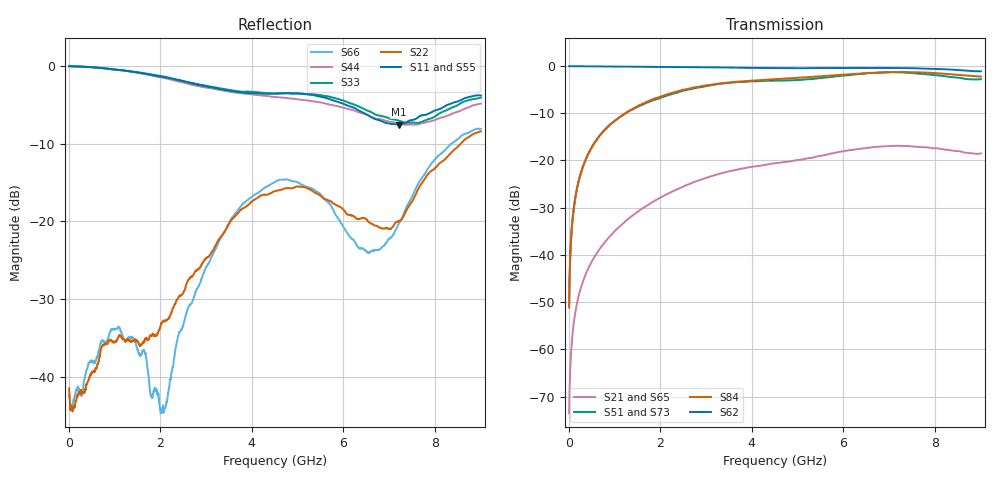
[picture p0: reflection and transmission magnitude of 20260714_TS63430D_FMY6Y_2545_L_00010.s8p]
# GHz S DB R 50
! CMT, SN0916, 25263762, 26.7.0
! Date: 15.07.2026 14:52:27
! Data: Format
! Freq S1.1:dB/Ang S1.2:dB/Ang S1.3:dB/Ang S1.4:dB/Ang S1.5:dB/Ang S1.6:dB/Ang S1.7:dB/Ang S1.8:dB/Ang
!  S2.1:dB/Ang S2.2:dB/Ang S2.3:dB/Ang S2.4:dB/Ang S2.5:dB/Ang S2.6:dB/Ang S2.7:dB/Ang S2.8:dB/Ang
!  S3.1:dB/Ang S3.2:dB/Ang S3.3:dB/Ang S3.4:dB/Ang S3.5:dB/Ang S3.6:dB/Ang S3.7:dB/Ang S3.8:dB/Ang
!  S4.1:dB/Ang S4.2:dB/Ang S4.3:dB/Ang S4.4:dB/Ang S4.5:dB/Ang S4.6:dB/Ang S4.7:dB/Ang S4.8:dB/Ang
!  S5.1:dB/Ang S5.2:dB/Ang S5.3:dB/Ang S5.4:dB/Ang S5.5:dB/Ang S5.6:dB/Ang S5.7:dB/Ang S5.8:dB/Ang
!  S6.1:dB/Ang S6.2:dB/Ang S6.3:dB/Ang S6.4:dB/Ang S6.5:dB/Ang S6.6:dB/Ang S6.7:dB/Ang S6.8:dB/Ang
!  S7.1:dB/Ang S7.2:dB/Ang S7.3:dB/Ang S7.4:dB/Ang S7.5:dB/Ang S7.6:dB/Ang S7.7:dB/Ang S7.8:dB/Ang
!  S8.1:dB/Ang S8.2:dB/Ang S8.3:dB/Ang S8.4:dB/Ang S8.5:dB/Ang S8.6:dB/Ang S8.7:dB/Ang S8.8:dB/Ang
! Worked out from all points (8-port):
!   2001 points, 10 MHz to 9 GHz, reference 50 ohm
!   strongest paths, dB at 10 MHz, 2.257 GHz, 4.505 GHz, 6.753 GHz, 9 GHz:
!     S62: -0.1, -0.3, -0.5, -0.5, -1.2
!     S84: -51.2, -5.7, -2.8, -1.4, -2.3
!     S51: -50.7, -6.0, -3.1, -1.5, -2.8
!     S73: -51.3, -6.1, -3.3, -1.7, -2.8
!     S21: -73.5, -26.6, -20.6, -17.2, -18.5
!     S65: -70.8, -26.7, -20.7, -17.2, -18.7
!   lowest |S11| = -7.5 dB at 7.202 GHz (marker M1), VSWR 2.45, Z = 21.2 - j9.17 ohm
!   |S11| at or under -10 dB: nowhere
